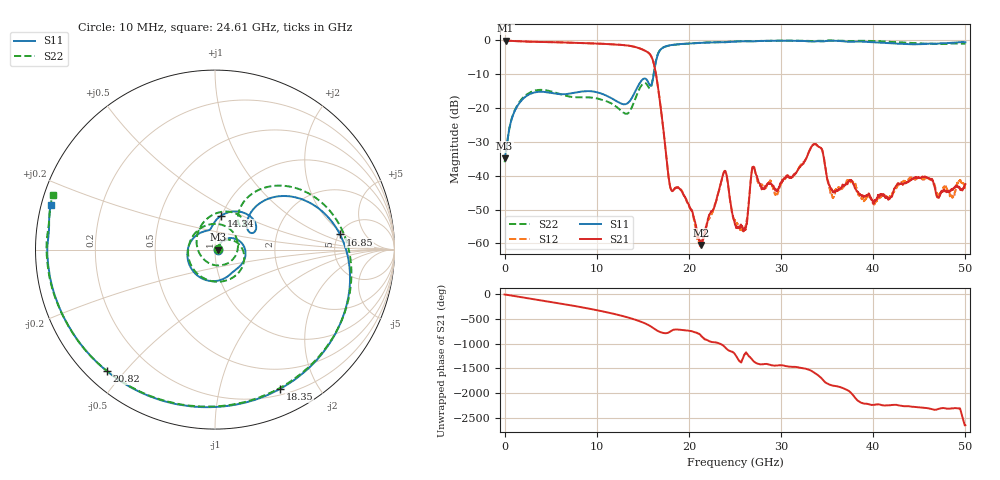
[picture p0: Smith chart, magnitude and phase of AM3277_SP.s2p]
!Keysight Technologies,N5245B,MY58422270,A.16.20.02
!Date: Tuesday, January 27, 2026 19:49:24
!Correction: S11(C  2-Port  )
!S21(C  2-Port  )
!S12(C  2-Port  )
!S22(C  2-Port  )
!S2P File: Measurements: S11, S21, S12, S22:
# Hz S  dB  R 50
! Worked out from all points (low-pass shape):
!   3201 points, 10 MHz to 50 GHz, reference 50 ohm
!   highest |S21| = -0.14 dB at 119.4 MHz (marker M1); lowest = -60.5 dB at 21.3 GHz (marker M2)
!   |S21| within 3 dB of the highest: start of sweep to 15.26 GHz
!   lowest |S11| = -34.9 dB at 10 MHz (marker M3), VSWR 1.04, Z = 51.8 + j0.00212 ohm
!   |S11| at or under -10 dB: start of sweep to 16.19 GHz
!   |S22| runs from -36.0 to -0.1 dB; largest |S21 - S12| = 0.014
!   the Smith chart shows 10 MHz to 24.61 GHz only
!   S11 on the Smith chart (normalised r, x): 10 MHz: 1.04, +0.00; 14.34 GHz: 0.99, +0.39; 16.85 GHz: 5.11, +1.70; 18.35 GHz: 0.26, -1.54; 20.82 GHz: 0.06, -0.45; 24.61 GHz: 0.03, +0.13
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1e7  -34.87 0.1  -0.14 -2.6  -0.13 -2.2  -36.03 17.2
1.193531e8  -33.38 17.3  -0.14 -4.6  -0.13 -4.3  -34.20 28.2
3.431191e9  -15.34 -5.8  -0.51 -103.0  -0.50 -103.1  -14.80 -38.0
5.946312e9  -15.93 -45.4  -0.65 179.5  -0.63 179.3  -15.82 -139.7
8.352081e9  -15.17 -85.5  -0.85 100.0  -0.83 99.7  -16.87 104.7
1.122651e10  -16.60 173.0  -1.15 -7.4  -1.13 -7.8  -18.19 -7.4
1.294491e10  -18.93 109.6  -1.47 -84.9  -1.45 -85.4  -21.46 -99.6
1.433526e10  -14.33 79.7  -2.14 -162.9  -2.12 -163.4  -16.22 119.8
1.556939e10  -12.32 24.2  -3.64 103.5  -3.61 103.1  -13.63 39.5
1.667854e10  -3.95 19.5  -14.42 -26.0  -14.39 -26.4  -3.79 24.5
1.685038e10  -3.08 6.9  -17.88 -40.6  -17.86 -41.0  -3.00 11.0
1.835008e10  -1.34 -65.1  -44.18 3.6  -44.13 1.4  -1.40 -64.5
2.081834e10  -0.86 -131.7  -55.35 -56.4  -57.35 -74.1  -0.85 -133.7
2.130262e10  -0.79 -141.5  -60.46 -116.0  -60.15 -119.5  -0.77 -144.0
2.380212e10  -0.62 175.7  -38.90 31.6  -38.94 30.2  -0.58 172.6
2.461445e10  -0.46 164.9  -49.80 -79.0  -49.64 -83.3  -0.41 161.5
2.5005e10  -0.42 159.6  -54.40 -134.7  -53.18 -131.7  -0.36 156.3
3.334708e10  -0.42 71.9  -31.29 -116.9  -31.27 -117.2  -0.30 74.1
3.559663e10  -0.18 49.6  -44.67 -50.3  -46.44 -48.5  -0.11 56.1
4.167354e10  -0.88 -35.2  -46.68 -89.1  -46.77 -91.3  -0.46 -0.7
4.517284e10  -1.20 -105.7  -40.61 -136.5  -40.78 -139.0  -0.96 -45.1
5e10  -0.62 172.9  -42.47 -136.2  -43.97 -153.5  -1.02 -128.1
